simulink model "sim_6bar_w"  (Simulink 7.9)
settings: Solver=ode45  StartTime=0.0  StopTime=10  RelTol=1e-3  AbsTol=1e-3
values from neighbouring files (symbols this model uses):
  g = 9806.65    [dyn_2dof.m]    (also in dyn_3dof.m; falling_sphere.m = 9.81; forward_2dof.m = 9.81)
  m = 1    [mechanical_system.m]
  s = Lv/norm(Lv)    [pkm1.m]
undefined symbols (not defined in the file or in its folder): cm, deg, kg, N
libraries: mblibv1 x27

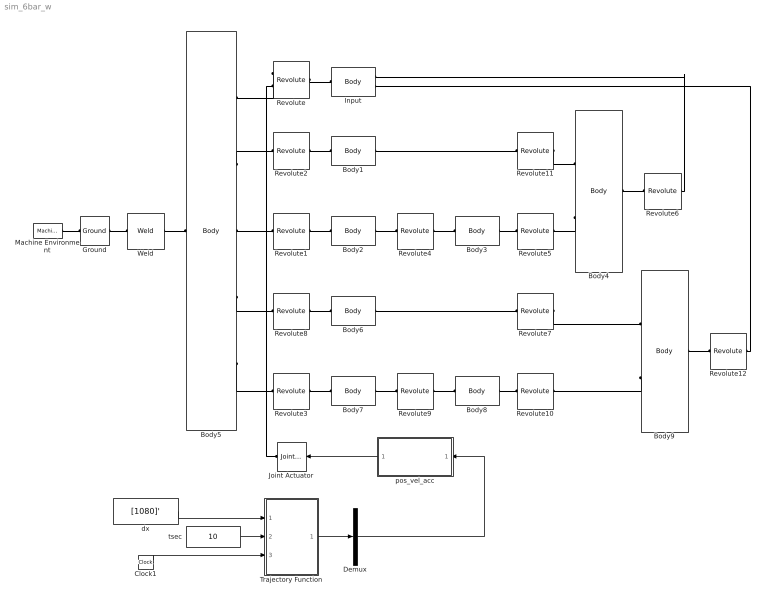
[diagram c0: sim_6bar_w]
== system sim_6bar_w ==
  Body1 : mblibv1/Bodies/Body  LConnTagsString=CS1  RConnTagsString=CS2  UpdateFromCAD=off  DialogClass=MechanicalBodyBlock  Mass=1.74  MassUnits=g  InertiaUnits=g*cm^2  Inertia=[2.0498 0 0; 0 2.0498 0; 0 0 0]  Shape=Cylinder  ShapeDims=[1 1]  ShapeUnits=m  ShapeUse=false  Density=1  DensityUnits=kg/m^3  DensityUse=false  GraphicsMode=MACHINE_DEFAULT  BodyColorSelMode=MACHINE_DEFAULT  BodyColor=[1 0 0]  AttachedToCS=CG  CG=Left$CG$[19.19/2 -32.22/2 0]$CS1$CS1$mm$[0 0 0]$Euler X-Y-Z$deg$WORLD$false$none  WorkingFrames=Left$CS1$[-52.5 0 0]$World$World$mm$[0 0 0]$Euler X-Y-Z$deg$WORLD$true$none#Right$CS2$[-33.31 -32.22 0]$World$World$mm$[0 0 0]$Euler X-Y-Z$deg$WORLD$true$none  CGPos=[19.19/2 -32.22/2 0]  CGRot=[0 0 0]  CS0Pos=[]  CS0Rot=[]  CS1Pos=[-52.5 0 0]  CS1Rot=[0 0 0]  CS2Pos=[-33.31 -32.22 0]  CS2Rot=[0 0 0]  CS3Pos=[]  CS3Rot=[]  CS4Pos=[]  CS4Rot=[]  CS5Pos=[]  CS5Rot=[]  CS6Pos=[]  CS6Rot=[]  CS7Pos=[]  CS7Rot=[]  CS8Pos=[]  CS8Rot=[]  CS9Pos=[]  CS9Rot=[]  CS10Pos=[]  CS10Rot=[]  CS11Pos=[]  CS11Rot=[]  CS12Pos=[]  CS12Rot=[]  CS13Pos=[]  CS13Rot=[]  CS14Pos=[]  CS14Rot=[]  CS15Pos=[]  CS15Rot=[]  CS16Pos=[]  CS16Rot=[]  CS17Pos=[]  CS17Rot=[]  CS18Pos=[]  CS18Rot=[]  CS19Pos=[]  CS19Rot=[]  CS20Pos=[]  CS20Rot=[]
  Body2 : mblibv1/Bodies/Body  LConnTagsString=CS1  RConnTagsString=CS2  UpdateFromCAD=off  DialogClass=MechanicalBodyBlock  Mass=9.65  MassUnits=g  InertiaUnits=g*cm^2  Inertia=[9.5332 0 0; 0 9.5332 0; 0 0 0]  Shape=Cylinder  ShapeDims=[1 1]  ShapeUnits=m  ShapeUse=false  Density=1  DensityUnits=kg/m^3  DensityUse=false  GraphicsMode=MACHINE_DEFAULT  BodyColorSelMode=MACHINE_DEFAULT  BodyColor=[1 0 0]  AttachedToCS=CG  CG=Left$CG$[-53.3/2 -27.55/2 0]$CS1$CS1$mm$[0 0 0]$Euler X-Y-Z$deg$WORLD$false$none  WorkingFrames=Left$CS1$[-52.50 0 0]$World$World$mm$[0 0 0]$Euler X-Y-Z$deg$WORLD$true$none#Right$CS2$[-105.8 -27.55 0]$World$World$mm$[0 0 0]$Euler X-Y-Z$deg$WORLD$true$none  CGPos=[-53.3/2 -27.55/2 0]  CGRot=[0 0 0]  CS0Pos=[]  CS0Rot=[]  CS1Pos=[-52.50 0 0]  CS1Rot=[0 0 0]  CS2Pos=[-105.8 -27.55 0]  CS2Rot=[0 0 0]  CS3Pos=[]  CS3Rot=[]  CS4Pos=[]  CS4Rot=[]  CS5Pos=[]  CS5Rot=[]  CS6Pos=[]  CS6Rot=[]  CS7Pos=[]  CS7Rot=[]  CS8Pos=[]  CS8Rot=[]  CS9Pos=[]  CS9Rot=[]  CS10Pos=[]  CS10Rot=[]  CS11Pos=[]  CS11Rot=[]  CS12Pos=[]  CS12Rot=[]  CS13Pos=[]  CS13Rot=[]  CS14Pos=[]  CS14Rot=[]  CS15Pos=[]  CS15Rot=[]  CS16Pos=[]  CS16Rot=[]  CS17Pos=[]  CS17Rot=[]  CS18Pos=[]  CS18Rot=[]  CS19Pos=[]  CS19Rot=[]  CS20Pos=[]  CS20Rot=[]
  Body3 : mblibv1/Bodies/Body  LConnTagsString=CS1  RConnTagsString=CS2  UpdateFromCAD=off  DialogClass=MechanicalBodyBlock  Mass=8.91  MassUnits=g  InertiaUnits=g*cm^2  Inertia=[9.6279 0 0; 0 9.6279 0; 0 0 0]  Shape=Cylinder  ShapeDims=[1 1]  ShapeUnits=m  ShapeUse=false  Density=1  DensityUnits=kg/m^3  DensityUse=false  GraphicsMode=MACHINE_DEFAULT  BodyColorSelMode=MACHINE_DEFAULT  BodyColor=[1 0 0]  AttachedToCS=CG  CG=Left$CG$[29.68/2 -49.83/2 0]$CS1$CS1$mm$[0 0 0]$Euler X-Y-Z$deg$WORLD$false$none  WorkingFrames=Left$CS1$[-105.8 -27.55 0]$World$World$mm$[0 0 0]$Euler X-Y-Z$deg$WORLD$true$none#Right$CS2$[-86.61 -59.77 0]$World$World$mm$[0 0 0]$Euler X-Y-Z$deg$WORLD$true$none#Right$CS3$[-76.12 -77.38 0]$World$World$mm$[0 0 0]$Euler X-Y-Z$deg$WORLD$false$none  CGPos=[29.68/2 -49.83/2 0]  CGRot=[0 0 0]  CS0Pos=[]  CS0Rot=[]  CS1Pos=[-105.8 -27.55 0]  CS1Rot=[0 0 0]  CS2Pos=[-86.61 -59.77 0]  CS2Rot=[0 0 0]  CS3Pos=[-76.12 -77.38 0]  CS3Rot=[0 0 0]  CS4Pos=[]  CS4Rot=[]  CS5Pos=[]  CS5Rot=[]  CS6Pos=[]  CS6Rot=[]  CS7Pos=[]  CS7Rot=[]  CS8Pos=[]  CS8Rot=[]  CS9Pos=[]  CS9Rot=[]  CS10Pos=[]  CS10Rot=[]  CS11Pos=[]  CS11Rot=[]  CS12Pos=[]  CS12Rot=[]  CS13Pos=[]  CS13Rot=[]  CS14Pos=[]  CS14Rot=[]  CS15Pos=[]  CS15Rot=[]  CS16Pos=[]  CS16Rot=[]  CS17Pos=[]  CS17Rot=[]  CS18Pos=[]  CS18Rot=[]  CS19Pos=[]  CS19Rot=[]  CS20Pos=[]  CS20Rot=[]
  Body4 : mblibv1/Bodies/Body  LConnTagsString=CS1|CS2  RConnTagsString=CS3  UpdateFromCAD=off  DialogClass=MechanicalBodyBlock  Mass=4.18  MassUnits=g  InertiaUnits=g*cm^2  Inertia=[8.1054 0 0; 0 8.1054 0; 0 0 0]  Shape=Cylinder  ShapeDims=[1 1]  ShapeUnits=m  ShapeUse=false  Density=1  DensityUnits=kg/m^3  DensityUse=false  GraphicsMode=MACHINE_DEFAULT  BodyColorSelMode=MACHINE_DEFAULT  BodyColor=[1 0 0]  AttachedToCS=CG  CG=Left$CG$[-86.61/2 -44.77/2 0]$CS3$CS3$mm$[0 0 0]$Euler X-Y-Z$deg$WORLD$false$none  WorkingFrames=Left$CS1$[-33.31 -32.22 0]$World$World$mm$[0 0 0]$Euler X-Y-Z$deg$WORLD$true$none#Left$CS2$[-86.61 -59.77 0]$World$World$mm$[0 0 0]$Euler X-Y-Z$deg$WORLD$true$none#Right$CS3$[0 -15 0]$World$World$mm$[0 0 0]$Euler X-Y-Z$deg$WORLD$true$none  CGPos=[-86.61/2 -44.77/2 0]  CGRot=[0 0 0]  CS0Pos=[]  CS0Rot=[]  CS1Pos=[-33.31 -32.22 0]  CS1Rot=[0 0 0]  CS2Pos=[-86.61 -59.77 0]  CS2Rot=[0 0 0]  CS3Pos=[0 -15 0]  CS3Rot=[0 0 0]  CS4Pos=[]  CS4Rot=[]  CS5Pos=[]  CS5Rot=[]  CS6Pos=[]  CS6Rot=[]  CS7Pos=[]  CS7Rot=[]  CS8Pos=[]  CS8Rot=[]  CS9Pos=[]  CS9Rot=[]  CS10Pos=[]  CS10Rot=[]  CS11Pos=[]  CS11Rot=[]  CS12Pos=[]  CS12Rot=[]  CS13Pos=[]  CS13Rot=[]  CS14Pos=[]  CS14Rot=[]  CS15Pos=[]  CS15Rot=[]  CS16Pos=[]  CS16Rot=[]  CS17Pos=[]  CS17Rot=[]  CS18Pos=[]  CS18Rot=[]  CS19Pos=[]  CS19Rot=[]  CS20Pos=[]  CS20Rot=[]
  Body5 : mblibv1/Bodies/Body  LConnTagsString=CS1  RConnTagsString=CS2|CS3|CS4|CS5|CS6  UpdateFromCAD=off  DialogClass=MechanicalBodyBlock  Mass=50  MassUnits=g  InertiaUnits=g*cm^2  Inertia=[0 0 0; 0 0 0; 0 0 0]  Shape=Cylinder  ShapeDims=[1 1]  ShapeUnits=m  ShapeUse=false  Density=1  DensityUnits=kg/m^3  DensityUse=false  GraphicsMode=MACHINE_DEFAULT  BodyColorSelMode=MACHINE_DEFAULT  BodyColor=[1 0 0]  AttachedToCS=CG  CG=Left$CG$[0 0 0]$World$World$mm$[0 0 0]$Euler X-Y-Z$deg$WORLD$false$none  WorkingFrames=Left$CS1$[0 0 0]$World$World$mm$[0 0 0]$Euler X-Y-Z$deg$WORLD$true$none#Right$CS2$[0 0 0]$World$World$mm$[0 0 0]$Euler X-Y-Z$deg$WORLD$true$none#Right$CS3$[-52.5 0 0]$World$World$mm$[0 0 0]$Euler X-Y-Z$deg$WORLD$true$none#Right$CS4$[-52.5 0 0]$World$World$mm$[0 0 0]$Euler X-Y-Z$deg$WORLD$true$none#Right$CS5$[52.5 0 0]$World$World$mm$[0 0 0]$Euler X-Y-Z$deg$WORLD$true$none#Right$CS6$[52.5 0 0]$Worl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  CGPos=[0 0 0]  CGRot=[0 0 0]  CS0Pos=[]  CS0Rot=[]  CS1Pos=[0 0 0]  CS1Rot=[0 0 0]  CS2Pos=[0 0 0]  CS2Rot=[0 0 0]  CS3Pos=[-52.5 0 0]  CS3Rot=[0 0 0]  CS4Pos=[-52.5 0 0]  CS4Rot=[0 0 0]  CS5Pos=[52.5 0 0]  CS5Rot=[0 0 0]  CS6Pos=[52.5 0 0]  CS6Rot=[0 0 0]  CS7Pos=[]  CS7Rot=[]  CS8Pos=[]  CS8Rot=[]  CS9Pos=[]  CS9Rot=[]  CS10Pos=[]  CS10Rot=[]  CS11Pos=[]  CS11Rot=[]  CS12Pos=[]  CS12Rot=[]  CS13Pos=[]  CS13Rot=[]  CS14Pos=[]  CS14Rot=[]  CS15Pos=[]  CS15Rot=[]  CS16Pos=[]  CS16Rot=[]  CS17Pos=[]  CS17Rot=[]  CS18Pos=[]  CS18Rot=[]  CS19Pos=[]  CS19Rot=[]  CS20Pos=[]  CS20Rot=[]
  Body6 : mblibv1/Bodies/Body  LConnTagsString=CS1  RConnTagsString=CS2  UpdateFromCAD=off  DialogClass=MechanicalBodyBlock  Mass=1.74  MassUnits=g  InertiaUnits=g*cm^2  Inertia=[2.0498 0 0; 0 2.0498 0; 0 0 0]  Shape=Cylinder  ShapeDims=[1 1]  ShapeUnits=m  ShapeUse=false  Density=1  DensityUnits=kg/m^3  DensityUse=false  GraphicsMode=MACHINE_DEFAULT  BodyColorSelMode=MACHINE_DEFAULT  BodyColor=[1 0 0]  AttachedToCS=CG  CG=Left$CG$[-19.19/2 -32.22/2 0]$CS1$CS1$mm$[0 0 0]$Euler X-Y-Z$deg$WORLD$false$none  WorkingFrames=Left$CS1$[52.5 0 0]$World$World$mm$[0 0 0]$Euler X-Y-Z$deg$WORLD$true$none#Right$CS2$[33.31 -32.22 0]$World$World$mm$[0 0 0]$Euler X-Y-Z$deg$WORLD$true$none  CGPos=[-19.19/2 -32.22/2 0]  CGRot=[0 0 0]  CS0Pos=[]  CS0Rot=[]  CS1Pos=[52.5 0 0]  CS1Rot=[0 0 0]  CS2Pos=[33.31 -32.22 0]  CS2Rot=[0 0 0]  CS3Pos=[]  CS3Rot=[]  CS4Pos=[]  CS4Rot=[]  CS5Pos=[]  CS5Rot=[]  CS6Pos=[]  CS6Rot=[]  CS7Pos=[]  CS7Rot=[]  CS8Pos=[]  CS8Rot=[]  CS9Pos=[]  CS9Rot=[]  CS10Pos=[]  CS10Rot=[]  CS11Pos=[]  CS11Rot=[]  CS12Pos=[]  CS12Rot=[]  CS13Pos=[]  CS13Rot=[]  CS14Pos=[]  CS14Rot=[]  CS15Pos=[]  CS15Rot=[]  CS16Pos=[]  CS16Rot=[]  CS17Pos=[]  CS17Rot=[]  CS18Pos=[]  CS18Rot=[]  CS19Pos=[]  CS19Rot=[]  CS20Pos=[]  CS20Rot=[]
  Body7 : mblibv1/Bodies/Body  LConnTagsString=CS1  RConnTagsString=CS2  UpdateFromCAD=off  DialogClass=MechanicalBodyBlock  Mass=9.65  MassUnits=g  InertiaUnits=g*cm^2  Inertia=[9.5332 0 0; 0 9.5332 0; 0 0 0]  Shape=Cylinder  ShapeDims=[1 1]  ShapeUnits=m  ShapeUse=false  Density=1  DensityUnits=kg/m^3  DensityUse=false  GraphicsMode=MACHINE_DEFAULT  BodyColorSelMode=MACHINE_DEFAULT  BodyColor=[1 0 0]  AttachedToCS=CG  CG=Left$CG$[53.3/2 -27.55/2 0]$CS1$CS1$mm$[0 0 0]$Euler X-Y-Z$deg$WORLD$false$none  WorkingFrames=Left$CS1$[52.50 0 0]$World$World$mm$[0 0 0]$Euler X-Y-Z$deg$WORLD$true$none#Right$CS2$[105.8 -27.55 0]$World$World$mm$[0 0 0]$Euler X-Y-Z$deg$WORLD$true$none  CGPos=[53.3/2 -27.55/2 0]  CGRot=[0 0 0]  CS0Pos=[]  CS0Rot=[]  CS1Pos=[52.50 0 0]  CS1Rot=[0 0 0]  CS2Pos=[105.8 -27.55 0]  CS2Rot=[0 0 0]  CS3Pos=[]  CS3Rot=[]  CS4Pos=[]  CS4Rot=[]  CS5Pos=[]  CS5Rot=[]  CS6Pos=[]  CS6Rot=[]  CS7Pos=[]  CS7Rot=[]  CS8Pos=[]  CS8Rot=[]  CS9Pos=[]  CS9Rot=[]  CS10Pos=[]  CS10Rot=[]  CS11Pos=[]  CS11Rot=[]  CS12Pos=[]  CS12Rot=[]  CS13Pos=[]  CS13Rot=[]  CS14Pos=[]  CS14Rot=[]  CS15Pos=[]  CS15Rot=[]  CS16Pos=[]  CS16Rot=[]  CS17Pos=[]  CS17Rot=[]  CS18Pos=[]  CS18Rot=[]  CS19Pos=[]  CS19Rot=[]  CS20Pos=[]  CS20Rot=[]
  Body8 : mblibv1/Bodies/Body  LConnTagsString=CS1  RConnTagsString=CS2  UpdateFromCAD=off  DialogClass=MechanicalBodyBlock  Mass=8.91  MassUnits=g  InertiaUnits=g*cm^2  Inertia=[9.6279 0 0; 0 9.6279 0; 0 0 0]  Shape=Cylinder  ShapeDims=[1 1]  ShapeUnits=m  ShapeUse=false  Density=1  DensityUnits=kg/m^3  DensityUse=false  GraphicsMode=MACHINE_DEFAULT  BodyColorSelMode=MACHINE_DEFAULT  BodyColor=[1 0 0]  AttachedToCS=CG  CG=Left$CG$[-29.68/2 -49.83/2 0]$CS1$CS1$mm$[0 0 0]$Euler X-Y-Z$deg$WORLD$false$none  WorkingFrames=Left$CS1$[105.8 -27.55 0]$World$World$mm$[0 0 0]$Euler X-Y-Z$deg$WORLD$true$none#Right$CS2$[86.61 -59.77 0]$World$World$mm$[0 0 0]$Euler X-Y-Z$deg$WORLD$true$none#Right$CS3$[76.12 -77.38 0]$World$World$mm$[0 0 0]$Euler X-Y-Z$deg$WORLD$false$none  CGPos=[-29.68/2 -49.83/2 0]  CGRot=[0 0 0]  CS0Pos=[]  CS0Rot=[]  CS1Pos=[105.8 -27.55 0]  CS1Rot=[0 0 0]  CS2Pos=[86.61 -59.77 0]  CS2Rot=[0 0 0]  CS3Pos=[76.12 -77.38 0]  CS3Rot=[0 0 0]  CS4Pos=[]  CS4Rot=[]  CS5Pos=[]  CS5Rot=[]  CS6Pos=[]  CS6Rot=[]  CS7Pos=[]  CS7Rot=[]  CS8Pos=[]  CS8Rot=[]  CS9Pos=[]  CS9Rot=[]  CS10Pos=[]  CS10Rot=[]  CS11Pos=[]  CS11Rot=[]  CS12Pos=[]  CS12Rot=[]  CS13Pos=[]  CS13Rot=[]  CS14Pos=[]  CS14Rot=[]  CS15Pos=[]  CS15Rot=[]  CS16Pos=[]  CS16Rot=[]  CS17Pos=[]  CS17Rot=[]  CS18Pos=[]  CS18Rot=[]  CS19Pos=[]  CS19Rot=[]  CS20Pos=[]  CS20Rot=[]
  Body9 : mblibv1/Bodies/Body  LConnTagsString=CS1|CS2  RConnTagsString=CS3  UpdateFromCAD=off  DialogClass=MechanicalBodyBlock  Mass=4.18  MassUnits=g  InertiaUnits=g*cm^2  Inertia=[8.1054 0 0; 0 8.1054 0; 0 0 0]  Shape=Cylinder  ShapeDims=[1 1]  ShapeUnits=m  ShapeUse=false  Density=1  DensityUnits=kg/m^3  DensityUse=false  GraphicsMode=MACHINE_DEFAULT  BodyColorSelMode=MACHINE_DEFAULT  BodyColor=[1 0 0]  AttachedToCS=CG  CG=Left$CG$[86.61/2 -44.77/2 0]$CS3$CS3$mm$[0 0 0]$Euler X-Y-Z$deg$WORLD$false$none  WorkingFrames=Left$CS1$[33.31 -32.22 0]$World$World$mm$[0 0 0]$Euler X-Y-Z$deg$WORLD$true$none#Left$CS2$[86.61 -59.77 0]$World$World$mm$[0 0 0]$Euler X-Y-Z$deg$WORLD$true$none#Right$CS3$[0 -15 0]$World$World$mm$[0 0 0]$Euler X-Y-Z$deg$WORLD$true$none  CGPos=[86.61/2 -44.77/2 0]  CGRot=[0 0 0]  CS0Pos=[]  CS0Rot=[]  CS1Pos=[33.31 -32.22 0]  CS1Rot=[0 0 0]  CS2Pos=[86.61 -59.77 0]  CS2Rot=[0 0 0]  CS3Pos=[0 -15 0]  CS3Rot=[0 0 0]  CS4Pos=[]  CS4Rot=[]  CS5Pos=[]  CS5Rot=[]  CS6Pos=[]  CS6Rot=[]  CS7Pos=[]  CS7Rot=[]  CS8Pos=[]  CS8Rot=[]  CS9Pos=[]  CS9Rot=[]  CS10Pos=[]  CS10Rot=[]  CS11Pos=[]  CS11Rot=[]  CS12Pos=[]  CS12Rot=[]  CS13Pos=[]  CS13Rot=[]  CS14Pos=[]  CS14Rot=[]  CS15Pos=[]  CS15Rot=[]  CS16Pos=[]  CS16Rot=[]  CS17Pos=[]  CS17Rot=[]  CS18Pos=[]  CS18Rot=[]  CS19Pos=[]  CS19Rot=[]  CS20Pos=[]  CS20Rot=[]
  Clock1 : Clock
  Demux : Demux  Outputs=1
  Ground : mblibv1/Bodies/Ground  UpdateFromCAD=off  LeftPortType=env  RightPortType=workingframe  PhysicalDomain=Mechanical  DialogClass=GroundBlock  CoordPosition=[0 0 0]  CoordPositionUnits=mm  StateVectorMgrId=1  MachineId=[1 0]  ShowEnvPort=on
  Input : mblibv1/Bodies/Body  LConnTagsString=CS1  RConnTagsString=CS2|CS3  UpdateFromCAD=off  DialogClass=MechanicalBodyBlock  Mass=1.77  MassUnits=g  InertiaUnits=g*cm^2  Inertia=[1.2556 0 0; 0 1.2556 0; 0 0 0]  Shape=Cylinder  ShapeDims=[1 1]  ShapeUnits=m  ShapeUse=false  Density=1  DensityUnits=kg/m^3  DensityUse=false  GraphicsMode=MACHINE_DEFAULT  BodyColorSelMode=MACHINE_DEFAULT  BodyColor=[1 0 0]  AttachedToCS=CG  CG=Left$CG$[0 -7.5 0]$CS1$CS1$mm$[0 0 0]$Euler X-Y-Z$deg$WORLD$false$none  WorkingFrames=Left$CS1$[0 0 0]$World$World$mm$[0 0 0]$Euler X-Y-Z$deg$WORLD$true$none#Right$CS2$[0 -15 0]$World$World$mm$[0 0 0]$Euler X-Y-Z$deg$WORLD$true$none#Right$CS3$[0 -15 0]$World$World$mm$[0 0 0]$Euler X-Y-Z$deg$WORLD$true$none  CGPos=[0 -7.5 0]  CGRot=[0 0 0]  CS0Pos=[]  CS0Rot=[]  CS1Pos=[0 0 0]  CS1Rot=[0 0 0]  CS2Pos=[0 -15 0]  CS2Rot=[0 0 0]  CS3Pos=[0 -15 0]  CS3Rot=[0 0 0]  CS4Pos=[]  CS4Rot=[]  CS5Pos=[]  CS5Rot=[]  CS6Pos=[]  CS6Rot=[]  CS7Pos=[]  CS7Rot=[]  CS8Pos=[]  CS8Rot=[]  CS9Pos=[]  CS9Rot=[]  CS10Pos=[]  CS10Rot=[]  CS11Pos=[]  CS11Rot=[]  CS12Pos=[]  CS12Rot=[]  CS13Pos=[]  CS13Rot=[]  CS14Pos=[]  CS14Rot=[]  CS15Pos=[]  CS15Rot=[]  CS16Pos=[]  CS16Rot=[]  CS17Pos=[]  CS17Rot=[]  CS18Pos=[]  CS18Rot=[]  CS19Pos=[]  CS19Rot=[]  CS20Pos=[]  CS20Rot=[]
  Joint Actuator : mblibv1/Sensors &  Actuators/Joint Actuator  UpdateFromCAD=off  PhysicalDomain=Mechanical  PortType=blob  ActuationStyle=Motion  AngleUnits=deg  ArcVelocityUnits=deg/s  ArcAccelerationUnits=deg/s^2  CoordPositionUnits=m  VelocityUnits=m/s  AccelerationUnits=m/s^2  ForceUnits=N  TorqueUnits=N*m  ActiveIO=on  Width=3  DialogClass=MechanicalActuatorBlock  Primitive=R1  ReferenceFrame=Absolute (World)
  Machine Environment : mblibv1/Bodies/Machine Environment  PortType=env  PhysicalDomain=Mechanical  DialogTemplateClass=MECH.MachineEnvironment  SyncWhenCopied=off  Gravity=[0 -9.81 0]  GravityUnits=m/s^2  GravityAsSignal=off  Dimensionality=Auto-detect  AnalysisType=Forward dynamics  LinearAssemblyTolerance=1e-3  LinearAssemblyToleranceUnits=m  AngularAssemblyTolerance=1e-3  AngularAssemblyToleranceUnits=rad  ConstraintSolverType=Stabilizing  ConstraintRelTolerance=1e-4  ConstraintAbsTolerance=1e-4  UseRobustSingularityHandling=off  RedundancyAnalysisToleranceType=Automatically select tolerance  RedundancyAnalysisTolerance=1e-14  StatePerturbationType=Fixed  PerturbationSize=1e-5  VisualizeMachine=on  BodyVisualizationType=Use model default body geometries  BodyColorSelMode=Use model default  DefaultBodyColor=[1 0 0]
  Revolute : mblibv1/Joints/Revolute  LConnTagsString=__newl0|SA1  RConnTagsString=__newr0  UpdateFromCAD=off  NumSAPorts=1  CutJoint=off  MarkAsCut=off  Primitives=prismatic  PrimitiveProps=R1$World$[0 0 1]$revolute  DialogClass=JointBlock  R1Axis=[0 0 1]
  Revolute{1..12} (12 alike) : mblibv1/Joints/Revolute  LConnTagsString=__newl0  RConnTagsString=__newr0  UpdateFromCAD=off  NumSAPorts=0  CutJoint=off  MarkAsCut=off  Primitives=prismatic  PrimitiveProps=R1$WORLD$[0 0 1]$revolute  DialogClass=JointBlock  R1Axis=[0 0 1]
  Trajectory Function : MATLAB Function  TreatAsAtomicUnit=on
  Weld : mblibv1/Joints/Weld  LConnTagsString=__newl0  RConnTagsString=__newr0  UpdateFromCAD=off  NumSAPorts=0  CutJoint=off  MarkAsCut=off  Primitives=weld  PrimitiveProps=W$WORLD$[0 0 0]$weld  DialogClass=JointBlock  WAxis=[0 0 0]
  dx : Constant  Value=[1080]'
  pos_vel_acc : Subsystem
  tsec : Constant  Value=10
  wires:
  Clock1/1 -> Trajectory Function/3(tout)
  tsec/1 -> Trajectory Function/2(tsec)
  dx/1 -> Trajectory Function/1(dx)
  Demux/1 -> pos_vel_acc/1(In1)
  Trajectory Function/1(xd) -> Demux/1
  pos_vel_acc/1(Motion1) -> Joint Actuator/1
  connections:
  Revolute/RConn1 -- Input/LConn1
  Revolute6/LConn1 -- Input/RConn1
  Revolute11/LConn1 -- Body4/LConn1
  Revolute6/RConn1 -- Body4/RConn1
  Revolute11/RConn1 -- Body1/RConn1
  Body1/LConn1 -- Revolute2/LConn1
  Body4/LConn2 -- Revolute5/LConn1
  Revolute5/RConn1 -- Body3/RConn1
  Body3/LConn1 -- Revolute4/LConn1
  Revolute4/RConn1 -- Body2/RConn1
  Body2/LConn1 -- Revolute1/LConn1
  Revolute/LConn1 -- Body5/RConn1
  Machine Environment/RConn1 -- Ground/LConn1
  Ground/RConn1 -- Weld/LConn1
  Weld/RConn1 -- Body5/LConn1
  Revolute/LConn2 -- Joint Actuator/RConn1
  Body5/RConn2 -- Revolute2/RConn1
  Body5/RConn3 -- Revolute1/RConn1
  Body6/LConn1 -- Revolute8/LConn1
  Body7/LConn1 -- Revolute3/LConn1
  Revolute7/RConn1 -- Body6/RConn1
  Body9/LConn2 -- Revolute10/LConn1
  Revolute10/RConn1 -- Body8/RConn1
  Revolute9/RConn1 -- Body7/RConn1
  Revolute12/RConn1 -- Body9/RConn1
  Body8/LConn1 -- Revolute9/LConn1
  Revolute7/LConn1 -- Body9/LConn1
  Body5/RConn4 -- Revolute8/RConn1
  Body5/RConn5 -- Revolute3/RConn1
  Revolute12/LConn1 -- Input/RConn2

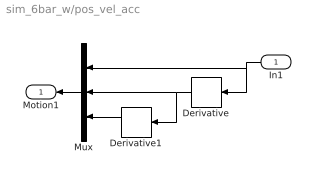
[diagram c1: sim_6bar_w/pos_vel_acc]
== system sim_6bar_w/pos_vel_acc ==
  In1 : Inport
  Derivative : Derivative
  Derivative1 : Derivative
  Mux : Mux  Inputs=3
  Motion1 : Outport
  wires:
  Derivative/1 -> Mux/2, Derivative1/1
  Derivative1/1 -> Mux/3
  In1/1 -> Mux/1, Derivative/1
  Mux/1 -> Motion1/1

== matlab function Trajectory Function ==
function xd = fcn(dx, tsec, tout)

MAX_CH=1;       % Two Actuators %
D2R=pi/180;

% Initializing Variables %
xd=zeros(MAX_CH,1);
x0=D2R*[0,0]';



    [c] = coeff_3rd(x0, zeros(MAX_CH,1), x0+dx, zeros(MAX_CH,1), tsec);
    for ch=1:MAX_CH
        xd(ch,1)=c(ch,1)+c(ch,2)*tout+c(ch,3)*tout^2+c(ch,4)*tout^3;    
    end

function [c] = coeff_3rd(sp, sv, ep, ev, tsec)
MAX_CH=1;
c=zeros(MAX_CH,4);
for ch=1:MAX_CH
    c(ch,1)=sp(ch,1);
    c(ch,2)=sv(ch,1);
    c(ch,3)=(3.0*(ep(ch,1)-sp(ch,1))-(2.0*sv(ch,1)+ev(ch,1))*tsec)/(tsec*tsec);
    c(ch,4)=(-2.0*(ep(ch,1)-sp(ch,1))+(sv(ch,1)+ev(ch,1))*tsec)/(tsec*tsec*tsec);
end
